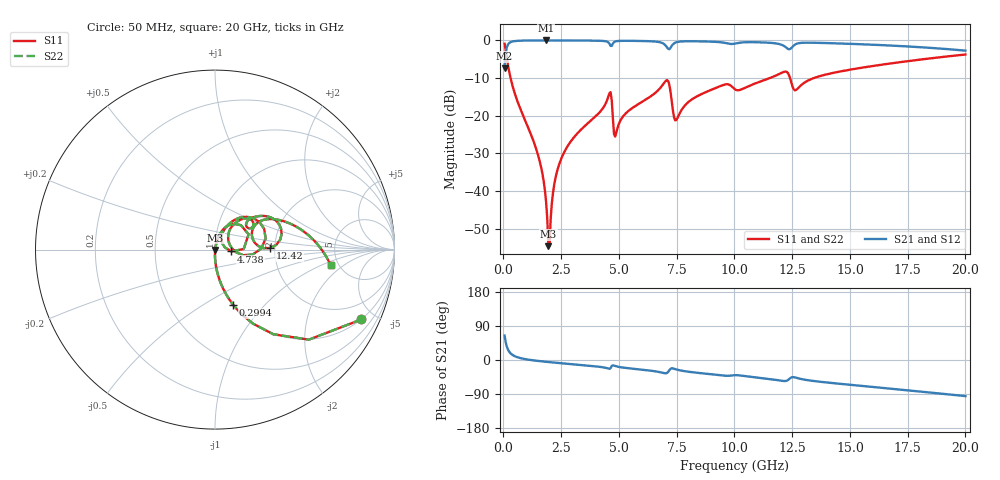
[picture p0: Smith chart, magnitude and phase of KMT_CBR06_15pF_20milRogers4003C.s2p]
! Data measured by Modelithics Inc. support@modelithics.com 813-866-6335
! KEMET CBR0603 15pF, Pad Width= 0.851mm, Pad Length= 0.64mm, Pad Gap= 0.62mm, 20mil Rogers 4003C substrate Data, January 2022
# hz S ma R 50
! 2 Port Network Data from SP1.SP block
! freq  magS11  angS11  magS21  angS21  magS12  angS12  magS22  angS22
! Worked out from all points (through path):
!   401 points, 50 MHz to 20 GHz, reference 50 ohm
!   highest |S21| = -0.01 dB at 1.845 GHz (marker M1); lowest = -7.4 dB at 50 MHz (marker M2)
!   group delay of S21, straight-line fit = 13.8 ps
!   lowest |S11| = -54.6 dB at 1.945 GHz (marker M3), VSWR 1.00, Z = 50.1 - j0.15 ohm
!   |S11| at or under -10 dB: 308.7 MHz to 11.53 GHz (11.22 GHz wide, 190 % of centre); 12.41 GHz to 13.43 GHz (1.026 GHz wide, 7.94 % of centre)
!   |S22| runs from -54.6 to -0.9 dB; largest |S21 - S12| = 0
!   S11 on the Smith chart (normalised r, x): 50 MHz: 0.99, -4.19; 299.4 MHz: 0.99, -0.68; 4.738 GHz: 1.20, -0.02; 12.42 GHz: 1.89, +0.04; 20 GHz: 4.31, -1.30
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5e7  0.9032 -25.5  0.4289 64.4  0.4289 64.4  0.9032 -25.5
2.99375e8  0.3251 -71.8  0.9451 18.1  0.9451 18.1  0.3251 -71.8
1.496375e9  0.03017 -90.4  0.9984 -2.5  0.9984 -2.5  0.03017 -90.4
1.695875e9  0.0164 -89.8  0.9987 -3.8  0.9987 -3.8  0.0164 -89.8
1.8455e9  0.007233 -85.2  0.9987 -4.8  0.9987 -4.8  0.007233 -85.2
1.94525e9  0.00186 -53.6  0.9987 -5.4  0.9987 -5.4  0.00186 -53.6
2.444e9  0.02419 78.4  0.9982 -8.2  0.9982 -8.2  0.02419 78.4
3.391625e9  0.06703 75.0  0.9957 -13.3  0.9957 -13.3  0.06703 75.0
4.588625e9  0.1985 43.2  0.904 -23.3  0.904 -23.3  0.1985 43.2
4.73825e9  0.09238 -6.4  0.9082 -13.9  0.9082 -13.9  0.09238 -6.4
4.887875e9  0.06026 52.0  0.9765 -16.8  0.9765 -16.8  0.06026 52.0
6.73325e9  0.224 52.4  0.9511 -31.6  0.9511 -31.6  0.224 52.4
7.13225e9  0.2888 12.4  0.771 -31.3  0.771 -31.3  0.2888 12.4
7.481375e9  0.08748 28.5  0.945 -24.8  0.945 -24.8  0.08748 28.5
8.478875e9  0.1877 52.6  0.972 -34.3  0.972 -34.3  0.1877 52.6
1.0025e10  0.2241 31.9  0.9075 -40.1  0.9075 -40.1  0.2241 31.9
1.18205e10  0.3445 32.5  0.91 -52.7  0.91 -52.7  0.3445 32.5
1.2419e10  0.3087 1.7  0.7713 -47.9  0.7713 -47.9  0.3087 1.7
1.266838e10  0.22 21.1  0.8953 -46.7  0.8953 -46.7  0.22 21.1
1.336662e10  0.3106 31.8  0.9324 -54.9  0.9324 -54.9  0.3106 31.8
1.670825e10  0.4921 13.1  0.8566 -75.4  0.8566 -75.4  0.4921 13.1
2e10  0.6503 -7.7  0.7317 -95.3  0.7317 -95.3  0.6503 -7.7
